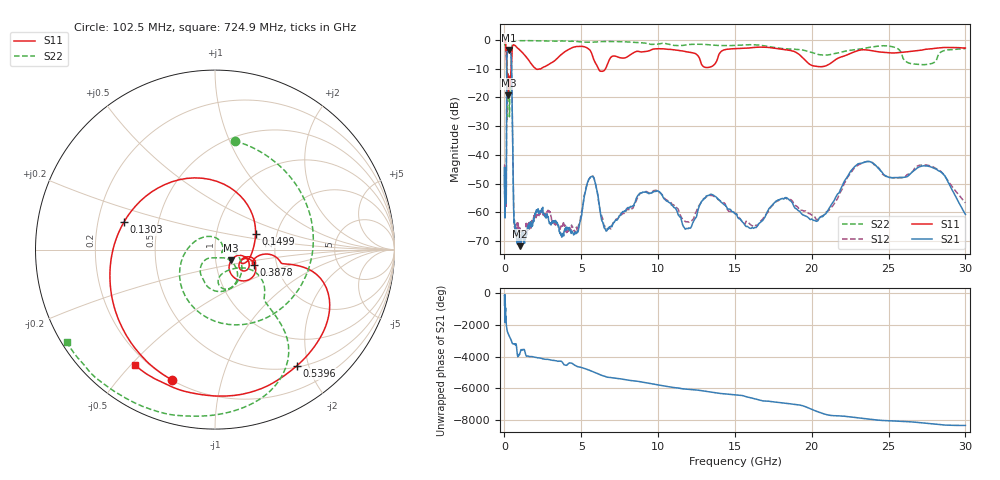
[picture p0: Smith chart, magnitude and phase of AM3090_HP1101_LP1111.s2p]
! Date/Time: Thu, Feb 28, 2019 2:08 PM
! Network Analyzer: Agilent Technologies E8364B Rev: A.07.50.67
! Sweep from 0.010 to 30.000 GHz, 1601 Points, Sweep Type: LOG
! Power Supply: 5.023 V, 0.002 A
# Hz S DB R 50
!freq MagS11 AngS11 MagS21 AngS21 MagS12 AngS12 MagS22 AngS22
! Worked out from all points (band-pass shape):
!   1601 points, 10 MHz to 30 GHz, reference 50 ohm
!   highest |S21| = -3.53 dB at 299 MHz (marker M1); lowest = -71.8 dB at 1.029 GHz (marker M2)
!   |S21| within 3 dB of the highest: 155.2 MHz to 443.6 MHz (288.4 MHz wide, 96.3 % of centre)
!   lowest |S11| = -19.3 dB at 253.4 MHz (marker M3), VSWR 1.24, Z = 59.5 - j7.22 ohm
!   |S11| at or under -10 dB: 144.1 MHz to 432.2 MHz (288 MHz wide, 100 % of centre); 2.035 GHz to 2.391 GHz (356.1 MHz wide, 16.1 % of centre); 6.107 GHz to 6.583 GHz (475.5 MHz wide, 7.49 % of centre)
!   |S22| runs from -27.8 to -0.2 dB; largest |S21 - S12| = 0.011
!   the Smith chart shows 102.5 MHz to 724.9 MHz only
!   S11 on the Smith chart (normalised r, x): 102.5 MHz: 0.20, -0.70; 130.3 MHz: 0.31, +0.13; 149.9 MHz: 1.55, +0.29; 387.8 MHz: 1.53, -0.28; 539.6 MHz: 0.52, -1.81; 724.9 MHz: 0.15, -0.51
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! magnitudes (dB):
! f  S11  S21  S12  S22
! 10 MHz  -0.3  -46.4  -51.0  -0.7
! 38.04 MHz  -0.4  -61.4  -59.1  -1.6
! 102.5 MHz  -2.3  -55.6  -52.6  -4.2
! 115 MHz  -3.3  -56.5  -57.5  -4.9
! 130.3 MHz  -5.5  -33.2  -32.9  -6.3
! 144.7 MHz  -10.3  -11.8  -11.7  -16.1
! 149.9 MHz  -12.3  -8.3  -8.2  -23.0
! 253.4 MHz  -19.3  -3.6  -3.5  -14.1
! 299 MHz  -13.4  -3.5  -3.5  -18.7
! 387.8 MHz  -12.6  -4.3  -4.3  -14.5
! 462 MHz  -7.6  -9.0  -9.0  -7.1
! 539.6 MHz  -2.0  -40.1  -39.8  -0.6
! 550.5 MHz  -1.9  -43.8  -43.8  -0.5
! 724.9 MHz  -2.1  -66.6  -65.9  -0.2
! 1.029 GHz  -3.7  -71.8  -66.7  -0.3
! 2.084 GHz  -10.2  -59.2  -61.1  -0.3
! 4.617 GHz  -2.4  -66.9  -66.2  -0.5
! 5.64 GHz  -4.3  -47.6  -47.5  -0.8
! 7.926 GHz  -6.1  -58.9  -59.5  -0.7
! 20.2 GHz  -9.1  -62.9  -61.6  -4.7
! 23.48 GHz  -3.5  -42.5  -42.5  -2.9
! 30 GHz  -2.8  -60.7  -56.7  -3.1
